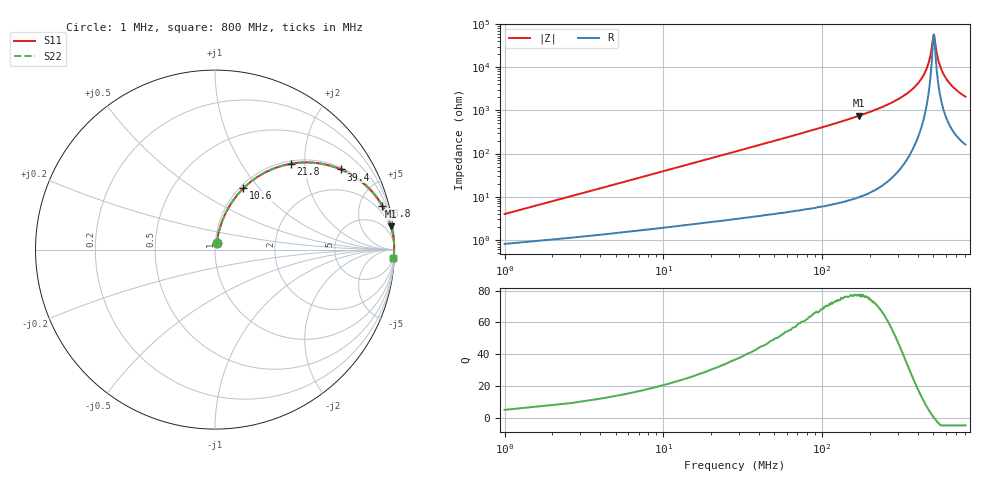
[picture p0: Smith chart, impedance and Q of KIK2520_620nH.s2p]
!version-2
!date-01.2022
!Series
# MHz S RI R 50
!Freq ReS11 ImS11 ReS21 ImS21 ReS12 ImS12 ReS22 ImS22
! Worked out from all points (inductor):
!   501 points, 1 MHz to 800 MHz, reference 50 ohm
!   read as one part in series: L = 620 nH near 4.2 MHz
!   highest Q = 77.3 at 171 MHz (marker M1), where L = 698 nH
!   self-resonance near 505 MHz
!   S11 on the Smith chart (normalised r, x): 1 MHz: 1.02, +0.08; 10.6 MHz: 1.04, +0.83; 21.8 MHz: 1.05, +1.70; 39.4 MHz: 1.07, +3.09; 93.8 MHz: 1.12, +7.57; 800 MHz: 4, -41
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1  0.00947 0.0383  0.9905 -0.0383  0.9905 -0.0383  0.00947 0.0383
5.8  0.0615 0.2089  0.9385 -0.2089  0.9385 -0.2089  0.0615 0.2089
10.6  0.1575 0.3413  0.8425 -0.3413  0.8425 -0.3413  0.1575 0.3413
21.8  0.4226 0.4784  0.5774 -0.4784  0.5774 -0.4784  0.4226 0.4784
39.4  0.7005 0.4467  0.2995 -0.4467  0.2995 -0.4467  0.7005 0.4467
61.8  0.8521 0.346  0.1479 -0.346  0.1479 -0.346  0.8521 0.346
93.8  0.9315 0.2451  0.0685 -0.2451  0.0685 -0.2451  0.9315 0.2451
135  0.9678 0.1699  0.0322 -0.1699  0.0322 -0.1699  0.9678 0.1699
171  0.9809 0.1306  0.0191 -0.1306  0.0191 -0.1306  0.9809 0.1306
268  0.9941 0.0683  0.00588 -0.0683  0.00588 -0.0683  0.9941 0.0683
401  0.9981 0.0238  0.00189 -0.0238  0.00189 -0.0238  0.9981 0.0238
435  0.9983 0.0155  0.00168 -0.0155  0.00168 -0.0155  0.9983 0.0155
467  0.9984 0.00825  0.00163 -0.00825  0.00163 -0.00825  0.9984 0.00825
483  0.9983 0.00484  0.00165 -0.00484  0.00165 -0.00484  0.9983 0.00484
505  0.9983 0.000254  0.00173 -0.000254  0.00173 -0.000254  0.9983 0.000254
510  0.9982 -0.000701  0.00175 0.000701  0.00175 0.000701  0.9982 -0.000701
524  0.9982 -0.00351  0.00184 0.00351  0.00184 0.00351  0.9982 -0.00351
534  0.9981 -0.00535  0.0019 0.00535  0.0019 0.00535  0.9981 -0.00535
551  0.998 -0.00863  0.00204 0.00863  0.00204 0.00863  0.998 -0.00863
583  0.9976 -0.0143  0.00236 0.0143  0.00236 0.0143  0.9976 -0.0143
667  0.9965 -0.028  0.00348 0.028  0.00348 0.028  0.9965 -0.028
800  0.994 -0.0475  0.00601 0.0475  0.00601 0.0475  0.994 -0.0475
